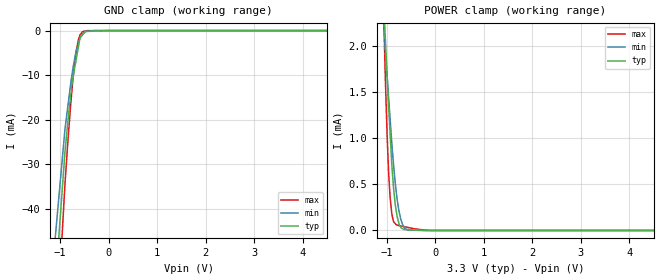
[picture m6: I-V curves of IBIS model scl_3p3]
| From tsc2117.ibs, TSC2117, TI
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|   scl_3p3 Model
[Model]   scl_3p3
Model_type   Input
Vinl = 0.99
Vinh = 2.31
|   typ   min   max
|   (nom PVT)   (fast PVT)   (slow PVT)
|C_comp from frequency sweep method (F=400KHz)
|Average
|C_comp   3.575e-12   3.526e-12   3.610e-12
|C_comp from LC tank measurement(L=1nH)
|Average
|Resonant Frequency(Hz)   4.770e+09   4.790e+09   4.760e+09
C_comp   1.114e-12   1.105e-12   1.119e-12
| Where nom  PVT is Nominal Process, 3.3V, 48C
|   Fast PVT is Strong Process,  3.6V, -40C
|   Slow PVT is Weak Process,   3V, 108C
[Model Spec]
|Subparameter   typ   min   max
Vinh   2.31   2.1   2.52
Vinl   0.99   0.9   1.08
[Voltage Range]   3.3   3   3.6
|Ambient Temperature   25   85   -40
|Junction Temperature
[Temperature Range]   48   108   -40
[Power Clamp Reference]   3.3   3   3.6
[GND Clamp Reference]   0   0   0
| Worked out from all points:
|   GND clamp passes 1 mA (typ) near -0.55 V on its own axis
|   POWER clamp passes 1 mA (typ) near -0.93 V on its own axis
[GND Clamp]
|   Voltage   I(typ)   I(min)   I(max)
-3.3V     -1.756A    -1.583A    -1.981A
-1.498V   -117.6mA   -94.96mA   -151.4mA
-897.6mV  -27.23mA   -22.13mA   -34.46mA
-788.4mV  -15.45mA   -12.65mA   -17.84mA
-745.8mV  -11.34mA   -9.432mA   -12.44mA
-698.4mV  -8.438mA   -6.377mA   -7.366mA
-622.8mV  -3.816mA   -2.95mA    -2.159mA
-590.7mV  -1.853mA   -1.714mA   -1.121mA
-532.8mV  -666.4uA   -905.1uA   -230.1uA
-474mV    -201.1uA   -197.3uA   -92.23uA
-285mV    -120.3uA   -2.039uA   -5.286uA
6.6V      0A         0A         0A
[POWER Clamp]
|   Voltage   I(typ)   I(min)   I(max)
-3.3V     32.35mA    22.57mA    56.44mA
-1.092V   2.8mA      2.46mA     2.906mA
-1.033V   2.101mA    1.972mA    1.686mA
-993.6mV  1.657mA    1.668mA    1.017mA
-964.8mV  1.359mA    1.451mA    640.5uA
-932.4mV  1.048mA    1.207mA    355.4uA
-896.4mV  705.6uA    935.8uA    174.6uA
-858mV    438.3uA    688.4uA    92.2uA
-788.7mV  152.2uA    339.5uA    59.13uA
-714mV    36.66uA    125.5uA    49.1uA
-643.5mV  10.58uA    34.75uA    41.33uA
6.6V      0A         0A         0A
